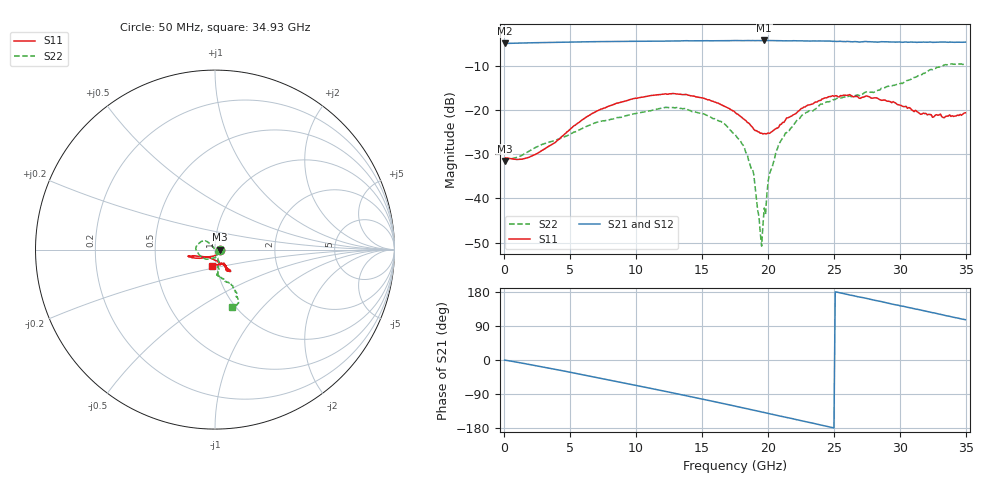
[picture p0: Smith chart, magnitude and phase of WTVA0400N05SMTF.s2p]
! 50 ohm 2-Port S-parameters measured by Modelithics Inc support@modelithics.com  Tampa, FL USA 813-866-6335 (February 2024)
! Smiths Interconnect,  4dB P/N: WTVA0400N05SMTF, Temperature: 0 C
! Board: 10 mil Rogers 4350B, Mounting Pad Dimensions: Length: 15 mils, Width: 25 mils, Gap: 40 mils.
# Hz S RI R 50
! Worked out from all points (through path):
!   352 points, 50 MHz to 34.93 GHz, reference 50 ohm
!   highest |S21| = -4.23 dB at 19.7 GHz (marker M1); lowest = -4.9 dB at 50 MHz (marker M2)
!   group delay of S21, straight-line fit = 20.5 ps
!   lowest |S11| = -31.5 dB at 50 MHz (marker M3), VSWR 1.05, Z = 52.7 - j0.0765 ohm
!   |S11| at or under -10 dB: start of sweep to end of sweep
!   |S22| runs from -50.8 to -9.5 dB; largest |S21 - S12| = 0.0039
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5e7  0.0266 -0.000725  0.5686 -0.00258  0.5685 -0.00273  0.0284 -0.000666
2.4885e9  0.00209 -0.032  0.5589 -0.1544  0.5587 -0.1543  0.01 -0.0369
5.8715e9  -0.0617 -0.0452  0.4662 -0.3665  0.4658 -0.3666  -0.0314 -0.0527
8.558e9  -0.1101 -0.0474  0.3278 -0.5013  0.3271 -0.5014  -0.0691 -0.0447
1.1742e10  -0.1449 -0.0378  0.1108 -0.5932  0.1099 -0.5932  -0.1037 -0.00598
1.5125e10  -0.1313 -0.0365  -0.1483 -0.5909  -0.1488 -0.5906  -0.0792 0.0437
1.7513e10  -0.0858 -0.0368  -0.3245 -0.5205  -0.3249 -0.52  -0.0353 0.0391
1.811e10  -0.07 -0.0384  -0.3634 -0.4917  -0.3638 -0.4911  -0.0246 0.0315
1.88065e10  -0.0491 -0.041  -0.4085 -0.4573  -0.4085 -0.4569  -0.0149 0.016
1.9304e10  -0.0344 -0.0447  -0.4372 -0.4285  -0.4377 -0.4276  -0.00479 0.00395
1.9503e10  -0.028 -0.0471  -0.4472 -0.4172  -0.4472 -0.4169  -0.00265 -0.00111
1.9702e10  -0.0216 -0.0497  -0.461 -0.4063  -0.4607 -0.4063  0.000258 -0.00779
1.98015e10  -0.0189 -0.0505  -0.4657 -0.398  -0.4653 -0.3982  0.000848 -0.00657
1.9901e10  -0.0162 -0.0516  -0.4702 -0.3924  -0.4698 -0.3926  0.00424 -0.0104
2.01e10  -0.0103 -0.0535  -0.4809 -0.3801  -0.4805 -0.3802  0.00477 -0.0183
2.07965e10  0.0124 -0.0627  -0.5134 -0.3314  -0.5136 -0.3307  0.0131 -0.0388
2.21895e10  0.0444 -0.0831  -0.5632 -0.2311  -0.5633 -0.2302  0.0216 -0.0743
2.33835e10  0.0632 -0.099  -0.5911 -0.14  -0.5909 -0.1397  0.0181 -0.0959
2.61695e10  0.0865 -0.1223  -0.591 0.0888  -0.5908 0.0891  0.0116 -0.1448
2.91545e10  0.063 -0.1087  -0.5086 0.3018  -0.5079 0.3025  0.0575 -0.1772
3.2438e10  0.0343 -0.0755  -0.3344 0.4794  -0.3329 0.48  0.1169 -0.261
3.49255e10  -0.0176 -0.0914  -0.1657 0.5644  -0.163 0.565  0.096 -0.3199
